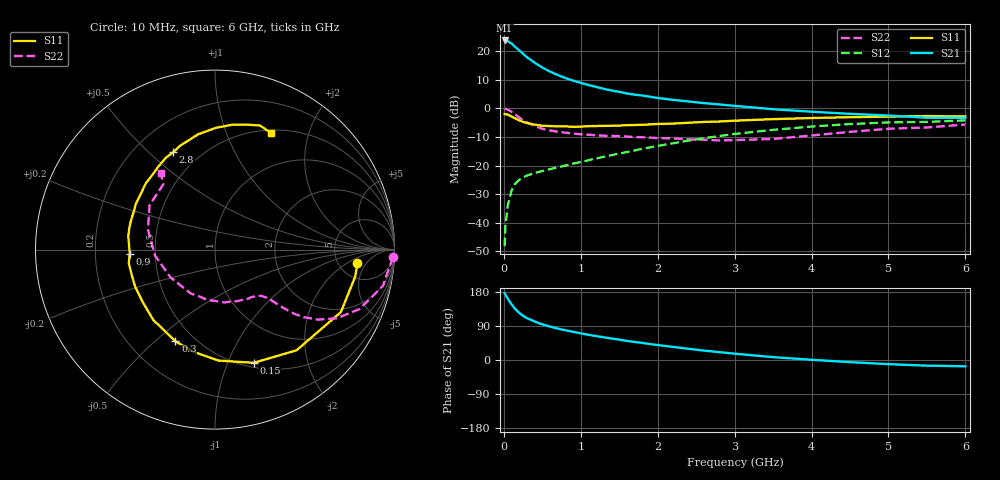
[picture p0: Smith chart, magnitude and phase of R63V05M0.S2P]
! SIEMENS Small Signal Semiconductors
! BFR193
! Si NPN RF Bipolar Junction Transistor in SOT23
! VCE = 3 V  IC = 5 mA
! Common Emitter S-Parameters:  May  1996
# GHz  S  MA  R  50
!  f  S11  S21  S12  S22
! GHz  MAG  ANG  MAG  ANG  MAG  ANG  MAG  ANG
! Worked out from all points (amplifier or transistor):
!   36 points, 10 MHz to 6 GHz, reference 50 ohm
!   highest |S21| = 23.8 dB at 10 MHz (marker M1)
!   |S21| within 3 dB of that: start of sweep to 180.3 MHz
!   unconditionally stable (mu >= 1): 881.7 MHz to 2.004 GHz
!   at 250 MHz: K = 0.43, MSG = 21.6 dB, |S12| = -24.1 dB
!   at 1.4 GHz: K = 1.07, MAG = 9.7 dB, |S12| = -16.4 dB
!   at 6 GHz: K = 0.96, MSG = 0.4 dB, |S12| = -4.2 dB
!   lowest NFmin = 1.20 dB at 450 MHz
!   S11 on the Smith chart (normalised r, x): 10 MHz: 7.53, -3.16; 150 MHz: 0.55, -1.25; 300 MHz: 0.39, -0.58; 900 MHz: 0.36, -0.02; 2.8 GHz: 0.36, +0.60; 6 GHz: 0.53, +1.45
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0.01  0.7974 -5.5  15.43 176.6  0.0039 90.1  0.9922 -2.5
0.02  0.7956 -10.9  15.19 172.7  0.0086 84.5  0.9799 -5.0
0.05  0.783 -26.4  14.94 162.5  0.0197 77.2  0.9572 -12.2
0.1  0.722 -51.0  13.63 147.1  0.0364 66.3  0.8716 -22.3
0.15  0.6667 -71.1  11.8 134.2  0.0486 58.3  0.7794 -29.4
0.2  0.6187 -88.2  10.38 124.3  0.0561 53.3  0.6938 -34.2
0.25  0.5812 -102.4  8.991 116.5  0.0621 49.8  0.6205 -37.3
0.3  0.556 -113.4  7.859 110.6  0.0669 48.3  0.5693 -39.0
0.4  0.5213 -131.3  6.315 101.5  0.0742 47.0  0.494 -40.6
0.5  0.4969 -144.9  5.18 94.0  0.0801 47.2  0.4412 -41.6
0.6  0.4905 -155.2  4.407 88.2  0.0865 48.7  0.4106 -42.2
0.7  0.4849 -163.7  3.841 82.9  0.0932 50.2  0.3921 -43.0
0.9  0.4757 -177.2  3.063 74.3  0.108 53.2  0.3639 -45.1
1.1  0.4886 171.5  2.568 66.5  0.1241 56.0  0.3465 -48.7
1.3  0.4948 161.9  2.197 59.9  0.1427 57.6  0.3331 -52.6
1.6  0.5093 150.1  1.824 50.3  0.1727 58.8  0.3212 -60.4
2.2  0.5428 130.1  1.412 34.5  0.2457 57.0  0.2991 -80.3
2.8  0.5904 113.3  1.174 20.7  0.3289 50.7  0.2753 -108.2
3.5  0.6494 98.3  0.968 7.6  0.4217 40.1  0.2921 -147.9
4.5  0.7025 82.1  0.803 -5.6  0.5326 23.2  0.3891 163.6
5.5  0.7354 70.0  0.687 -14.9  0.5809 6.1  0.4641 128.3
6  0.7211 64.5  0.683 -16.6  0.618 1.1  0.5225 125.4
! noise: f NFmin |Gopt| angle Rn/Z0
0.45  1.2  0.26  102  0.14
0.9  1.25  0.38  145  0.12
1.8  2.05  0.56  -161  0.12
